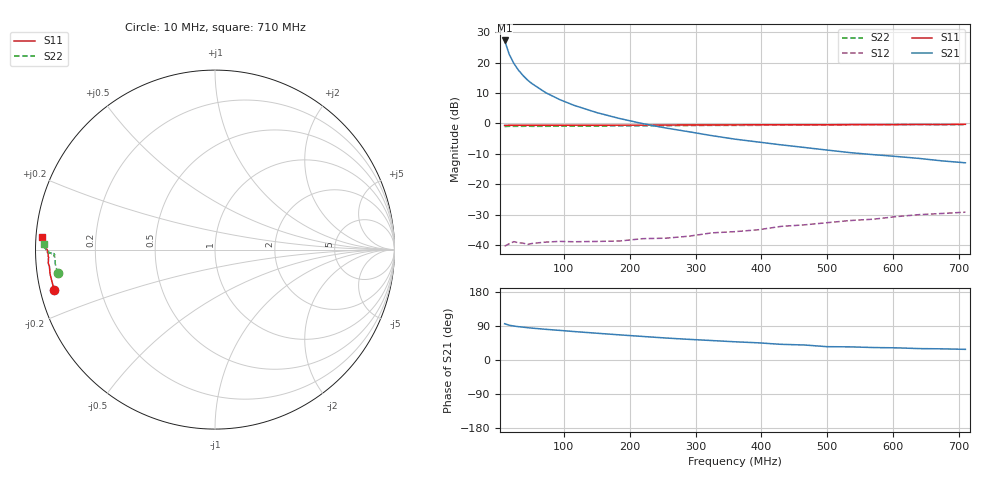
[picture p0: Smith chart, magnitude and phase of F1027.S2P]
! Date: Fri Jul 21 10:18:01 1995
# MHZ S MA R 50
!  POLYFET RF DEVICES
!  F1027 (Each Side)
!  S PARAMETERS
!  VDS=28V, IDQ=1.20mA
!  FREQ  S11MAG  S11ANG  S21MAG  S21ANG  S12MAG  S12ANG  S22MAG  S22ANG
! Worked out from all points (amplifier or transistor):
!   27 points, 10 MHz to 710 MHz, reference 50 ohm
!   highest |S21| = 27.2 dB at 10 MHz (marker M1)
!   |S21| within 3 dB of that: start of sweep to 14.59 MHz
!   unconditionally stable (mu >= 1): 223.7 MHz to 410.9 MHz
!   at 38 MHz: K = 0.24, MSG = 27.5 dB, |S12| = -39.4 dB
!   at 255 MHz: K = 1.10, MAG = 16.2 dB, |S12| = -37.7 dB
!   at 710 MHz: K = 0.74, MSG = 8.1 dB, |S12| = -29.2 dB
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10  0.9242 -165.9  23.03 95.7  0.00958 6.4  0.8855 -171.4
17  0.929 -171.7  13.6 91.8  0.0105 8.7  0.8941 -175.1
24  0.9273 -174.2  9.676 89.6  0.01136 7.2  0.8926 -176.3
31  0.9323 -175.4  7.49 87.9  0.01092 9.1  0.8935 -177.1
38  0.9295 -176.4  6.107 86.7  0.01074 9.4  0.8936 -177.3
45  0.9297 -176.8  5.131 85.3  0.01024 6.6  0.8982 -177.8
52  0.9281 -177.2  4.463 84.1  0.01063 11.0  0.8929 -178.2
73  0.9306 -178.0  3.167 80.9  0.01119 12.6  0.8948 -178.3
94  0.9295 -178.8  2.45 78.1  0.01148 15.9  0.8966 -178.5
115  0.9338 -179.0  1.985 75.1  0.01132 20.3  0.9045 -178.6
150  0.9316 -179.4  1.502 70.7  0.01146 24.5  0.9025 -178.6
185  0.9341 -179.5  1.199 66.3  0.01166 29.1  0.9087 -178.7
220  0.9355 180.0  0.9888 62.1  0.01273 38.5  0.9106 -178.6
255  0.9395 179.8  0.8382 58.0  0.01297 45.7  0.9125 -178.8
290  0.9419 179.4  0.7274 54.5  0.01397 46.4  0.9207 -178.8
325  0.9411 178.9  0.6276 51.3  0.01586 51.9  0.9257 -178.8
360  0.9438 178.8  0.55 48.1  0.0166 57.4  0.925 -179.1
395  0.9481 178.5  0.4937 45.3  0.0178 59.3  0.9277 -179.4
430  0.9479 178.4  0.4436 41.3  0.02026 66.7  0.9404 -179.5
500  0.9474 177.8  0.3637 35.2  0.02329 64.5  0.9428 179.9
605  0.9533 176.7  0.2857 32.1  0.02928 70.6  0.9536 179.1
710  0.9645 175.7  0.2248 28.1  0.03467 75.8  0.9519 178.1
